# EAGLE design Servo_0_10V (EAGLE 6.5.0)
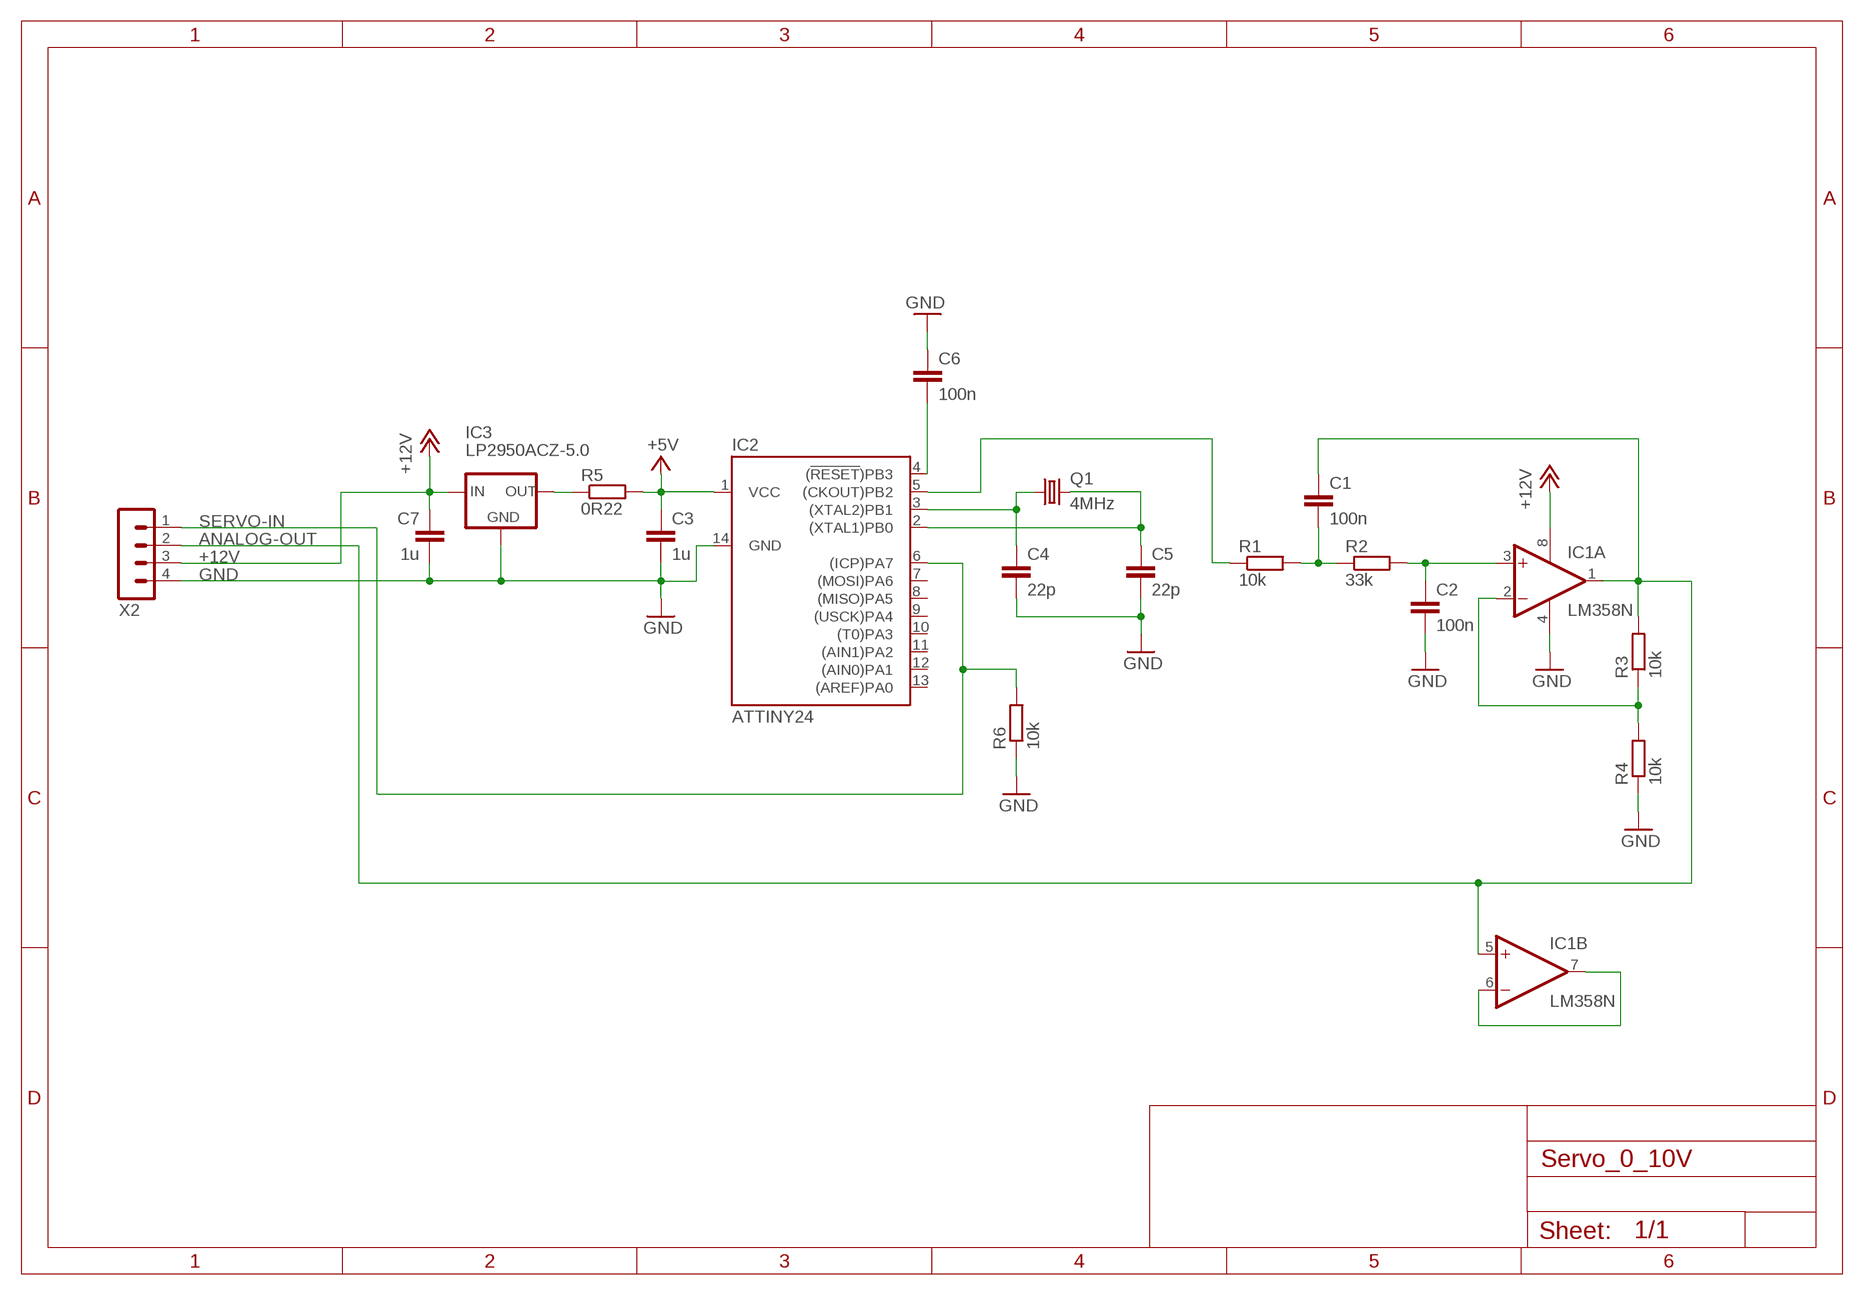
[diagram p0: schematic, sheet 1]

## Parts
C1  100n  C-EU025-024X044  [C025-024X044]
C2  100n  C-EU025-024X044  [C025-024X044]
C3  1u  C-EU050-024X044  [C050-024X044]
C4  22p  C-EU025-024X044  [C025-024X044]
C5  22p  C-EU025-024X044  [C025-024X044]
C6  100n  C-EU025-024X044  [C025-024X044]
C7  1u  C-EU025-024X044  [C025-024X044]
IC1  LM358N  [DIL08]
IC2  ATTINY24  [DIL14]
IC3  LP2950ACZ-5.0  [TO92]
Q1  4MHz  CRYSTALHC49U-V  [HC49U-V]
R1  10k  R-EU_0207/10  [0207/10]
R2  33k  R-EU_0207/10  [0207/10]
R3  10k  R-EU_0207/10  [0207/10]
R4  10k  R-EU_0207/10  [0207/10]
R5  0R22  R-EU_0207/10  [0207/10]
R6  10k  R-EU_0207/10  [0207/10]
X2  MA04-1  [MA04-1]

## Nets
+5V: C3.1 IC2.1(VCC) R5.2
+12V: C7.1 IC1.8(P:V+) IC3.3(IN) X2.3
ANALOG-OUT: C1.1 IC1.1(A:OUT) IC1.5(B:+IN) R3.2 X2.2
GND: C2.2 C3.2 C4.2 C5.2 C6.1 C7.2 IC1.4(P:V-) IC2.14(GND) IC3.2(GND) R4.1 R6.1 X2.4
N$1: IC1.6(B:-IN) IC1.7(B:OUT)
N$2: C1.2 R1.2 R2.1
N$3: C2.1 IC1.3(A:+IN) R2.2
N$4: IC1.2(A:-IN) R3.1 R4.2
N$5: IC3.1(OUT) R5.1
N$8: C4.1 IC2.3((XTAL2)PB1) Q1.1
N$9: C5.1 IC2.2((XTAL1)PB0) Q1.2
N$11: IC2.5((CKOUT)PB2) R1.1
N$12: C6.2 IC2.4((!RESET!)PB3)
SERVO-IN: IC2.6((ICP)PA7) R6.2 X2.1
Unconnected: IC2.7((MOSI)PA6) IC2.8((MISO)PA5) IC2.9((USCK)PA4) IC2.10((T0)PA3) IC2.11((AIN1)PA2) IC2.12((AIN0)PA1) IC2.13((AREF)PA0)

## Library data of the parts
C1-C7 = rcl:C-EU: CAPACITOR, European symbol
IC1 = linear:LM358: OP AMP also LM158; LM258; LM2904 Source: http://cache.national.com/ds/LM/LM158.pdf
IC2 = brunner:ATTINY24
IC3 = v-reg:LP2950?*: Source: http://cache.national.com/ds/LP/LP2950.pdf
Q1 = crystal:CRYSTAL: CRYSTAL; OC_FARNELL: 1666969; OC_NEWARK: unknown
R1-R6 = rcl:R-EU_: RESISTOR, European symbol
X2 = con-lstb:MA04-1: PIN HEADER; OC_FARNELL: unknown; OC_NEWARK: unknown

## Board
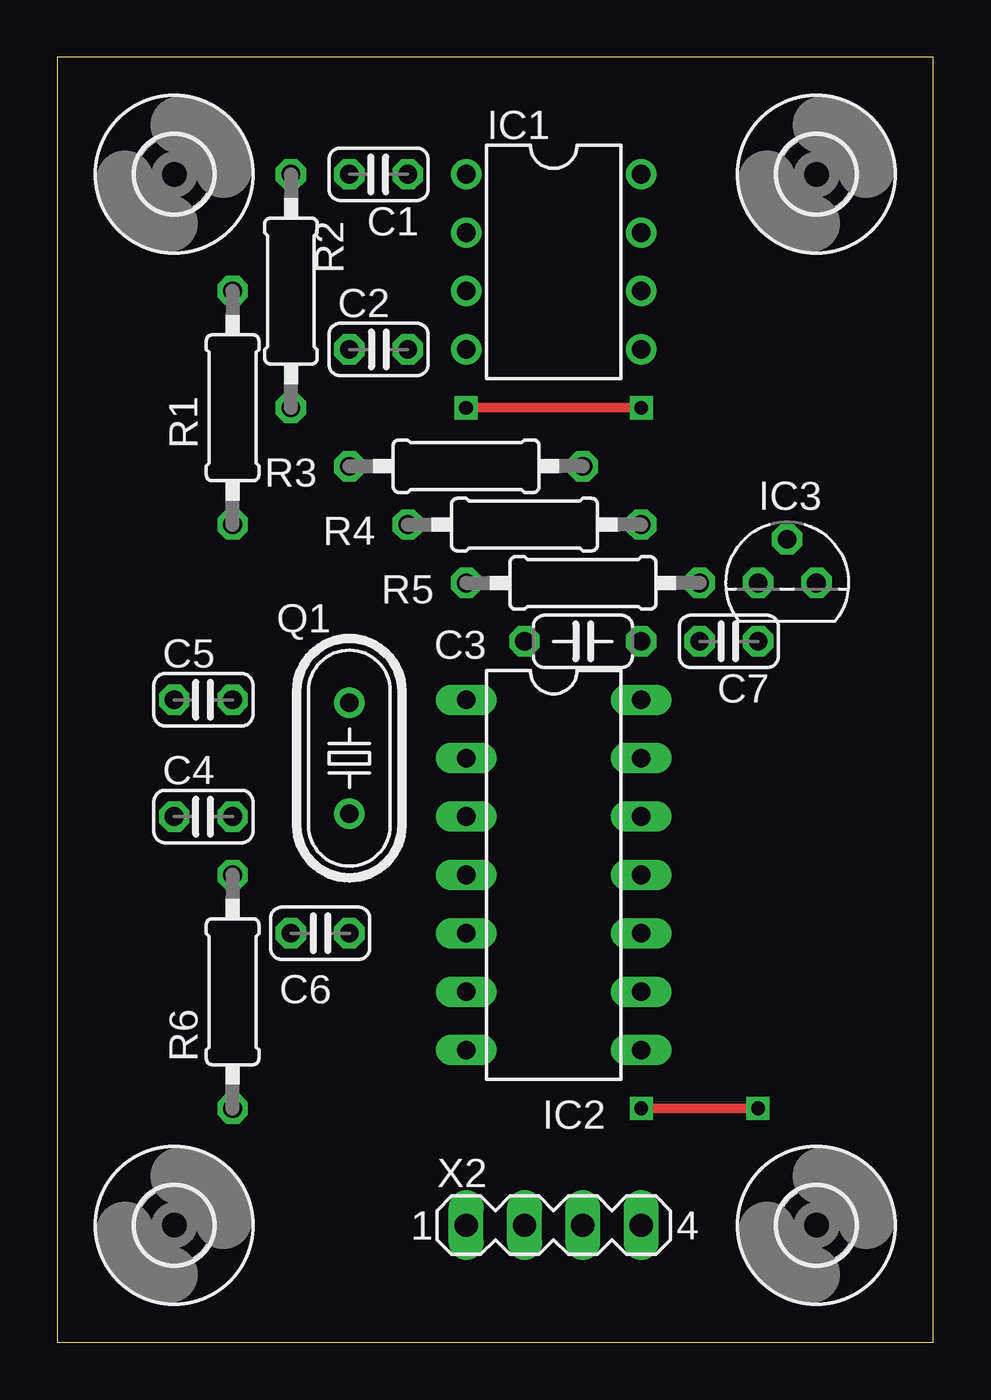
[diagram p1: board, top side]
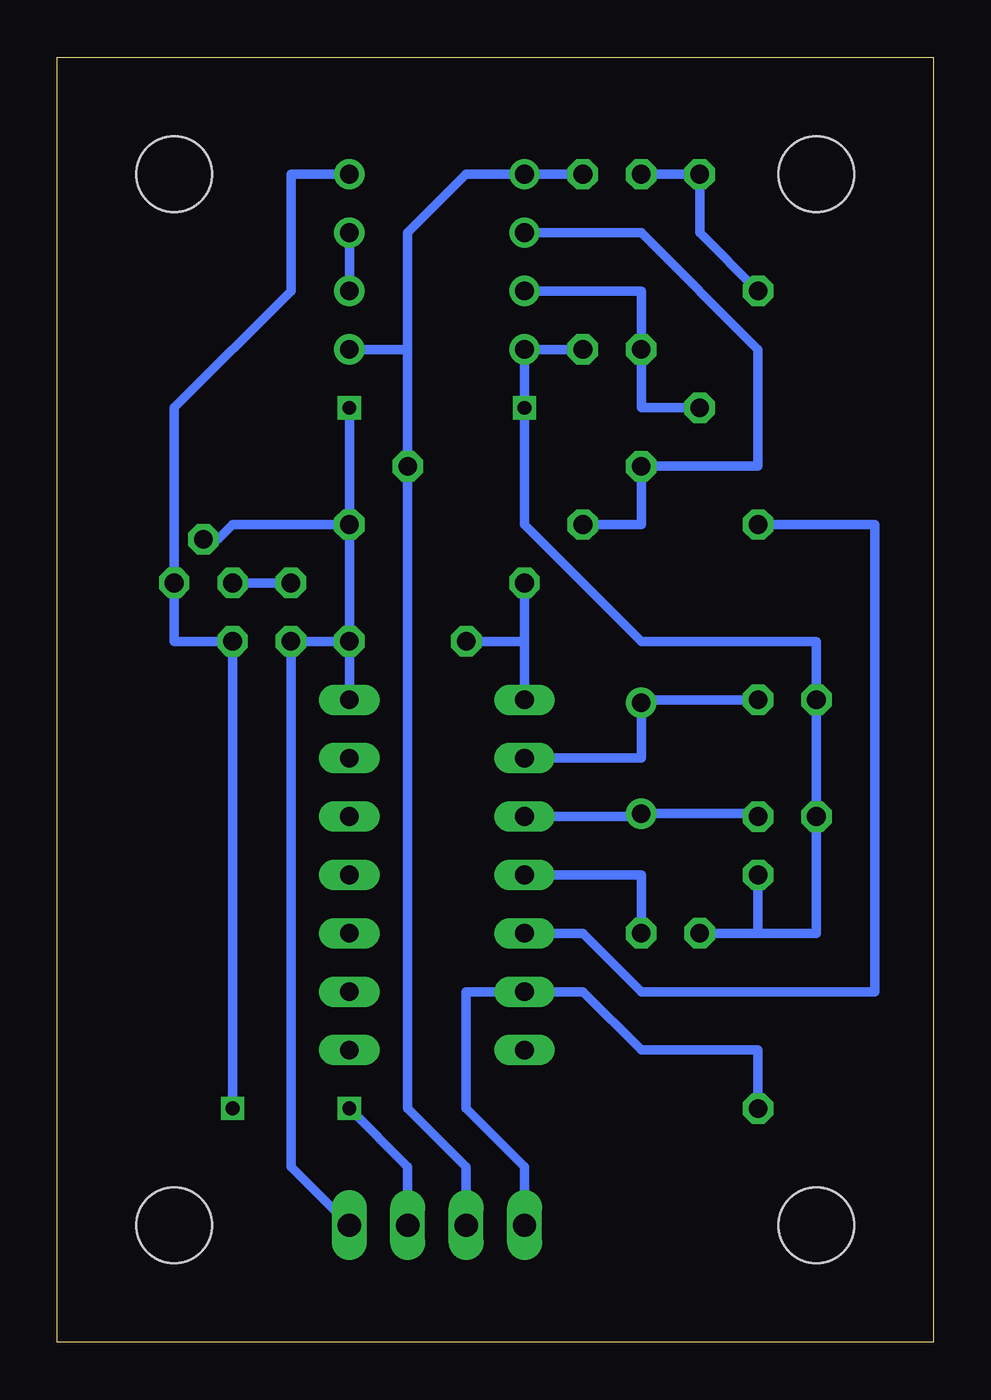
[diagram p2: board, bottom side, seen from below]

Size 38.1 x 55.88 mm. Coordinates in mm from the lower left corner, seen from the top.
Outline: 0,0 38.1,0 38.1,55.88 0,55.88 0,0
Copper layers (1*16): Top 0.035mm / dielectric 1.5mm / Bottom 0.035mm
Design rules "default *": minimum track width 10mil, minimum drill 0.6mm, track to track 8mil, track to pad 8mil, pad to pad 8mil, via to via 8mil, smd to smd 8mil, copper to edge 40mil, drill to drill 8mil, minimum pad ring 10mil, minimum via ring 8mil, stop-mask expansion 4mil, vias tented up to drill 0mil, thermal gap 10mil

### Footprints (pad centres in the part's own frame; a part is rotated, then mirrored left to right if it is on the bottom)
C025-024X044 = drill 0.813 octagon: 1 -1.27,0; 2 1.27,0
C050-024X044 = drill 0.813 octagon: 1 -2.54,0; 2 2.54,0
DIL08 = drill 0.813 pad 1.27: 1 -3.81,-3.81; 2 -1.27,-3.81; 3 1.27,-3.81; 4 3.81,-3.81; 5 3.81,3.81; 6 1.27,3.81; 7 -1.27,3.81; 8 -3.81,3.81
DIL14 = drill 0.813 long: 1 -7.62,-3.81; 2 -5.08,-3.81; 3 -2.54,-3.81; 4 0,-3.81; 5 2.54,-3.81; 6 5.08,-3.81; 7 7.62,-3.81; 8 7.62,3.81; 9 5.08,3.81; 10 2.54,3.81; 11 0,3.81; 12 -2.54,3.81; 13 -5.08,3.81; 14 -7.62,3.81
TO92 = drill 0.813 octagon: 1 -1.27,0; 2 0,1.905; 3 1.27,0
HC49U-V = drill 0.813: 1 -2.413,0; 2 2.413,0
0207/10 = drill 0.813 octagon: 1 -5.08,0; 2 5.08,0
3,3 = hole 3.3: 0,0
MA04-1 = drill 1.016 long: 1 -3.81,0; 2 -1.27,0; 3 1.27,0; 4 3.81,0

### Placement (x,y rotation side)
C1  13.97,50.8 180 top
C2  13.97,43.18 0 top
C3  22.86,30.48 0 top
C4  6.35,22.86 180 top
C5  6.35,27.94 180 top
C6  11.43,17.78 0 top
C7  29.21,30.48 180 top
IC1  21.59,46.99 270 top
IC2  21.59,20.32 270 top
IC3  31.75,33.02 0 top
Q1  12.7,25.4 90 top
R1  7.62,40.64 90 top
R2  10.16,45.72 270 top
R3  17.78,38.1 0 top
R4  20.32,35.56 180 top
R5  22.86,33.02 180 top
R6  7.62,15.24 270 top
U$1  [3,3]  5.08,5.08 0 top
U$2  [3,3]  33.02,50.8 0 top
U$3  [3,3]  33.02,5.08 0 top
U$4  [3,3]  5.08,50.8 0 top
U$5  [A4P-LOC]  not placed on the board
X2  21.59,5.08 0 top

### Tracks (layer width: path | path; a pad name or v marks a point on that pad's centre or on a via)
+5V
  Bottom 0.406: IC2.1 17.78,30.48 | 17.78,30.48 R5.2 | C3.1 17.78,30.48
+12V  (via drill 0.6)
  Top 0.406: v25.4,10.16 v30.48,10.16
  Bottom 0.406: IC1.8 27.94,50.8 27.94,45.72 33.02,40.64 IC3.3 33.02,30.48 C7.1 v30.48,10.16 | X2.3 22.86,7.62 v25.4,10.16
ANALOG-OUT
  Bottom 0.406: C1.1 IC1.1 20.32,50.8 22.86,48.26 22.86,43.18 | X2.2 20.32,7.62 22.86,10.16 R3.2 22.86,43.18 | IC1.5 22.86,43.18
GND  (via drill 0.6)
  Top 0.406: v25.4,40.64 v17.78,40.64
  Bottom 0.406: C2.2 IC1.4 v17.78,40.64 17.78,35.56 12.7,30.48 5.08,30.48 C5.2 C4.2 5.08,17.78 7.62,17.78 | C6.1 7.62,17.78 | C3.2 R4.1 | R4.1 v25.4,40.64 | C3.2 IC2.14 | X2.4 27.94,7.62 C7.2 C3.2 | IC3.2 31.11,34.92 30.48,35.56 R4.1 | R6.1 7.62,17.78
N$1
  Bottom 0.406: IC1.6 IC1.7
N$2
  Bottom 0.406: C1.2 R2.1 10.16,48.26 R1.2
N$3
  Bottom 0.406: IC1.3 12.7,45.72 C2.1 12.7,40.64 R2.2
N$4
  Bottom 0.406: IC1.2 12.7,48.26 7.62,43.18 7.62,38.1 R3.1 12.7,35.56 R4.2
N$5
  Bottom 0.406: R5.1 IC3.1
N$8
  Bottom 0.406: IC2.3 12.83,22.86 Q1.1 7.75,22.99 C4.1
N$9
  Bottom 0.406: C5.1 12.7,27.94 Q1.2 12.7,25.4 IC2.2
N$11
  Bottom 0.406: IC2.5 15.24,17.78 12.7,15.24 2.54,15.24 2.54,35.56 R1.1
N$12
  Bottom 0.406: IC2.4 12.7,20.32 C6.2
SERVO-IN
  Bottom 0.406: X2.1 17.78,7.62 20.32,10.16 20.32,15.24 IC2.6 15.24,15.24 12.7,12.7 7.62,12.7 R6.2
